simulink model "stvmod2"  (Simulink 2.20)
settings: Solver=FixedStepDiscrete  StartTime=0.0  StopTime=800  MaxStep=0.1  RelTol=1e-3  AbsTol=1e-6
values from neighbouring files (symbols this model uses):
  b = 0.5    [demo_stvmod.m]

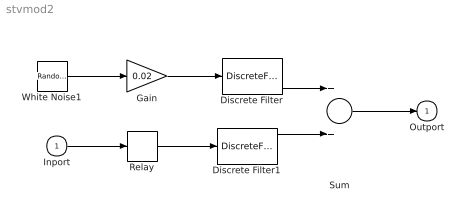
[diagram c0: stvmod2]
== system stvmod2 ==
  Inport : Inport  Port=1  PortWidth=-1  SampleTime=-1
  Discrete Filter : DiscreteFilter  Numerator=[1]  Denominator=[1 -0.9]  SampleTime=-1
  Discrete Filter1 : DiscreteFilter  Numerator=[b]  Denominator=[1 -0.9]  SampleTime=1
  Gain : Gain  Gain=0.02
  Relay : Relay  OnSwitchValue=0  OffSwitchValue=0  OnOutputValue=rele_up  OffOutputValue=rele_down
  Sum : Sum  Inputs=++
  White Noise1 : RandomNumber  Mean=0  Variance=0.02  Seed=201  SampleTime=0
  Outport : Outport  Port=1  InitialOutput=0
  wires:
  Gain/1 -> Discrete Filter/1
  White Noise1/1 -> Gain/1
  Relay/1 -> Discrete Filter1/1
  Discrete Filter1/1 -> Sum/2
  Discrete Filter/1 -> Sum/1
  Inport/1 -> Relay/1
  Sum/1 -> Outport/1
